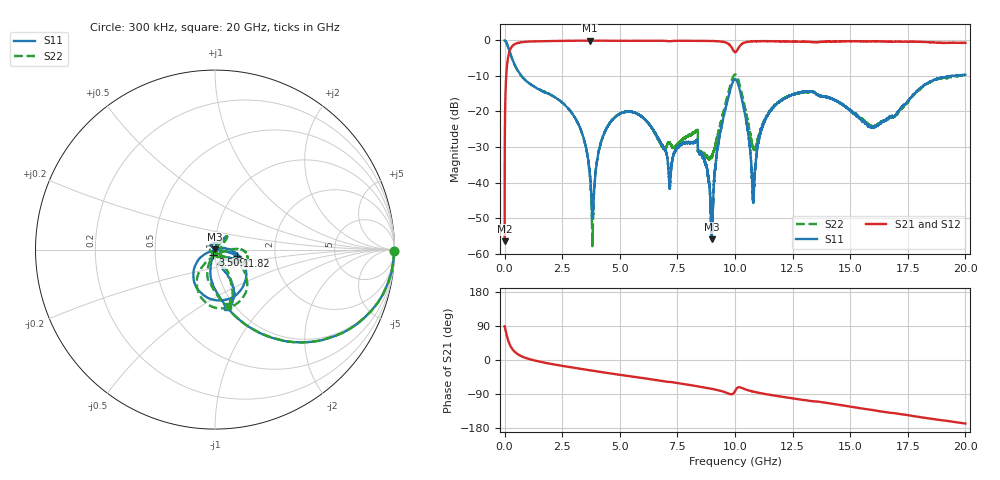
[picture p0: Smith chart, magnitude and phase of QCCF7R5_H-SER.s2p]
!{QCCF7R5}
!Johanson Technology Inc.
!www.johansontechnology.com
!Test Board Conditions:
!Substrate Type  RO4350B
!Substrate Thickness  10 mil
!Substrate Dk  3.66
!TL Type: GCPW
!TL Trace Width  21 mil
!TL Gap  20 mil
!Electrode orientation  Horizontal
!DUT TOPOLOGY	SERIES
!Mounting Pad LxW  16x21 mil
! Created Sat Jan  9 18:16:08 2021
# hz S ma R 50
! 2 Port Network Data from SP1.SP block
! freq  magS11  angS11  magS21  angS21  magS12  angS12  magS22  angS22
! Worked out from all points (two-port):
!   20001 points, 300 kHz to 20 GHz, reference 50 ohm
!   highest |S21| = -0.05 dB at 3.686 GHz (marker M1); lowest = -56.6 dB at 300 kHz (marker M2)
!   |S21| within 3 dB of the highest: 214.7 MHz to 9.954 GHz (9.739 GHz wide, 192 % of centre); 10.07 GHz to end of sweep
!   lowest |S11| = -56.0 dB at 8.983 GHz (marker M3), VSWR 1.00, Z = 49.9 + j0.129 ohm
!   |S11| at or under -10 dB: 731 MHz to 19.37 GHz (18.64 GHz wide, 185 % of centre); 19.4952 GHz to 19.49895 GHz (3.742 MHz wide, 0.0192 % of centre); 19.50769 GHz to 19.51197 GHz (4.282 MHz wide, 0.0219 % of centre)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
!   |S22| runs from -57.9 to 0.0 dB; largest |S21 - S12| = 0.015
!   S11 on the Smith chart (normalised r, x): 300 kHz: open; 3.509 GHz: 0.98, -0.06; 11.82 GHz: 1.28, -0.10; 20 GHz: 0.91, -0.65
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300000  0.9986 -0.4  0.001482 89.4  0.001437 91.0  0.9986 -0.5
1.113e8  0.8835 -29.0  0.4644 60.7  0.4641 60.8  0.8829 -28.9
2.993e8  0.583 -57.3  0.8041 32.1  0.8052 32.1  0.5829 -57.1
3.3343e9  0.05244 -107.5  0.993 -23.6  0.9931 -23.6  0.05242 -114.9
3.5093e9  0.03347 -107.1  0.993 -25.3  0.9935 -25.3  0.03302 -115.8
3.6863e9  0.01471 -102.2  0.9945 -27.0  0.9935 -27.0  0.01376 -114.4
3.8313e9  0.003502 -5.9  0.9934 -28.3  0.9932 -28.3  0.0023 14.4
4.1823e9  0.03661 55.1  0.9925 -31.7  0.9926 -31.6  0.03723 53.9
4.9623e9  0.09093 50.6  0.9882 -38.8  0.9881 -38.7  0.0918 50.3
6.6673e9  0.04164 52.1  0.9896 -53.7  0.9902 -53.7  0.04002 24.5
7.1753e9  0.008153 108.5  0.9746 -57.9  0.9739 -57.8  0.03614 -54.7
8.2863e9  0.03738 84.8  0.9864 -68.4  0.9856 -68.4  0.05267 -47.3
8.9833e9  0.00159 125.8  0.981 -75.9  0.9817 -75.8  0.02282 -90.7
9.3363e9  0.04592 11.0  0.9698 -80.8  0.9713 -80.7  0.06195 -37.3
1.00003e10  0.2856 -78.3  0.6836 -82.2  0.6819 -82.1  0.3311 -76.9
1.04563e10  0.08363 -153.0  0.9426 -77.5  0.9421 -77.5  0.1044 -126.5
1.07953e10  0.005524 -77.9  0.9724 -83.3  0.9723 -83.3  0.02982 -77.8
1.11553e10  0.05704 -8.0  0.9777 -88.1  0.9769 -87.9  0.05973 -6.1
1.18223e10  0.1292 -16.8  0.9721 -95.0  0.9751 -94.9  0.13 1.5
1.33343e10  0.1907 -26.2  0.9503 -108.5  0.9508 -108.5  0.1897 -20.6
1.66673e10  0.07979 -73.8  0.9622 -138.4  0.9541 -138.8  0.08213 -59.7
2e10  0.3273 -78.9  0.9258 -167.8  0.9172 -167.6  0.3226 -77.3
